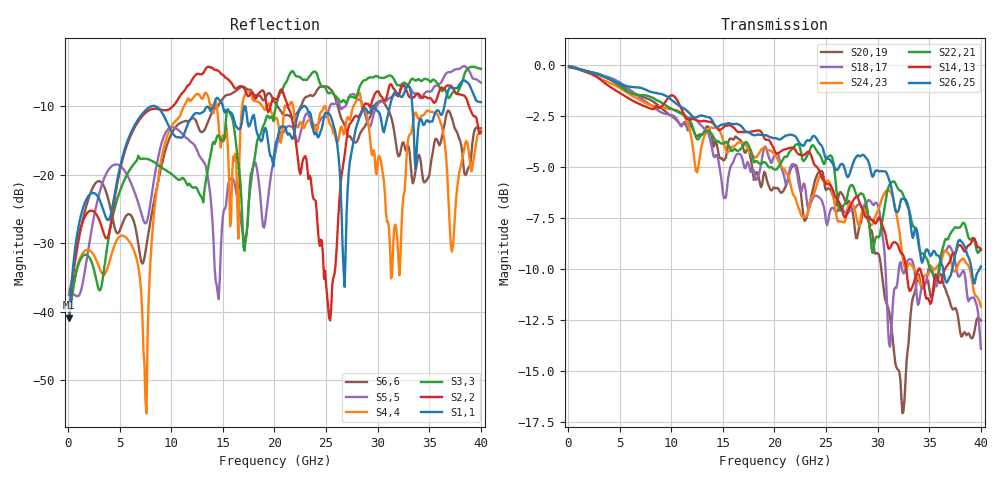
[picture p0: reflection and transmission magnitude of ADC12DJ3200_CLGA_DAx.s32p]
! Touchstone file
! Texas Instruments 4/21/2021
! ADC12DJ3200QML-SP
! Package-type  CLGA [BGA]
! pins/pkg drawing  196-pin ZMX
! CLGA Ceramic Package without columns (ceramic land grid array)
! High-speed serialized data output for channel A, lane 0-7
# GHZ S MA R 50.000000
! Port[1] = DA0N_BGA_F14
! Port[2] = DA0N_DIE_22
! Port[3] = DA0P_BGA_E14
! Port[4] = DA0P_DIE_21
! Port[5] = DA1N_BGA_D14
! Port[6] = DA1N_DIE_24
! Port[7] = DA1P_BGA_C14
! Port[8] = DA1P_DIE_23
! Port[9] = DA2N_BGA_A13
! Port[10] = DA2N_DIE_26
! Port[11] = DA2P_BGA_A12
! Port[12] = DA2P_DIE_25
! Port[13] = DA3N_BGA_A11
! Port[14] = DA3N_DIE_28
! Port[15] = DA3P_BGA_A10
! Port[16] = DA3P_DIE_27
! Port[17] = DA4N_BGA_F13
! Port[18] = DA4N_DIE_30
! Port[19] = DA4P_BGA_E13
! Port[20] = DA4P_DIE_29
! Port[21] = DA5N_BGA_D13
! Port[22] = DA5N_DIE_32
! Port[23] = DA5P_BGA_C13
! Port[24] = DA5P_DIE_31
! Port[25] = DA6N_BGA_B13
! Port[26] = DA6N_DIE_34
! Port[27] = DA6P_BGA_B12
! Port[28] = DA6P_DIE_33
! Port[29] = DA7N_BGA_B11
! Port[30] = DA7N_DIE_36
! Port[31] = DA7P_BGA_B10
! Port[32] = DA7P_DIE_35
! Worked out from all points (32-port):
!   400 points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, 100 MHz to 40 GHz, reference 50 ohm
!   strongest paths, dB at 100 MHz, 10.1 GHz, 20.1 GHz, 30.1 GHz, 40 GHz:
!     S26,25: -0.1, -1.7, -3.6, -5.2, -9.9
!     S14,13: -0.1, -1.5, -4.3, -7.5, -9.1
!     S22,21: -0.1, -2.2, -5.1, -8.4, -9.0
!     S24,23: -0.1, -2.2, -4.4, -7.0, -11.8
!     S18,17: -0.1, -2.5, -4.4, -7.0, -13.9
!     S20,19: -0.1, -2.5, -6.0, -9.3, -12.5
!   lowest |S11| = -40.9 dB at 100 MHz (marker M1), VSWR 1.02, Z = 50.8 - j0.36 ohm
!   |S11| at or under -10 dB: start of sweep to 8.166 GHz; 8.368 GHz to 14.12 GHz (5.751 GHz wide, 51.2 % of centre); 22.92 GHz to 29.54 GHz (6.619 GHz wide, 25.2 % of centre)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
